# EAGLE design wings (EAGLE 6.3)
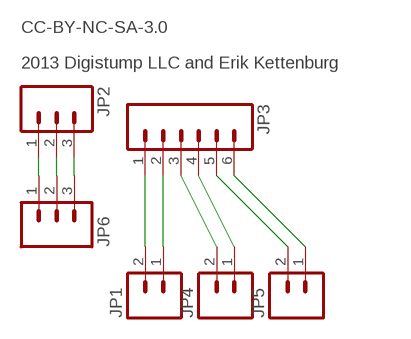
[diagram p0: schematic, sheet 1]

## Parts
JP1  M023.5MM  [SCREWTERMINAL-3.5MM-2]
JP2  M03PTH  [1X03]
JP3  M06SIP  [1X06]
JP4  M023.5MM  [SCREWTERMINAL-3.5MM-2]
JP5  M023.5MM  [SCREWTERMINAL-3.5MM-2]
JP6  M03SCREW  [SCREWTERMINAL-3.5MM-3]

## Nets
N$1: JP1.1 JP3.2
N$2: JP1.2 JP3.1
N$3: JP3.4 JP4.1
N$4: JP3.3 JP4.2
N$5: JP3.6 JP5.1
N$6: JP3.5 JP5.2
N$7: JP2.1 JP6.1
N$8: JP2.2 JP6.2
N$9: JP2.3 JP6.3

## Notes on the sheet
- CC-BY-NC-SA-3.0
- 2013 Digistump LLC and Erik Kettenburg

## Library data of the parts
JP1 JP4 JP5 = SparkFun:M02: Header 2
JP2 JP6 = SparkFun:M03: Header 3 Standard 3-pin 0.1" header. Use with straight break away headers (SKU : PRT-00116), right angle break away headers (PRT-00553), swiss pins (PRT-00743), machine pins (PRT-00117), and female headers (PRT-00115). Molex polarized connector foot print use with SKU : PRT-08232 with associated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
JP3 = SparkFun:M06: Header 6 Standard 6-pin 0.1" header. Use with straight break away headers (SKU : PRT-00116), right angle break away headers (PRT-00553), swiss pins (PRT-00743), machine pins (PRT-00117), and female headers (PRT-00115). Molex polarized connector foot print use with SKU : PRT-08094 with associated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

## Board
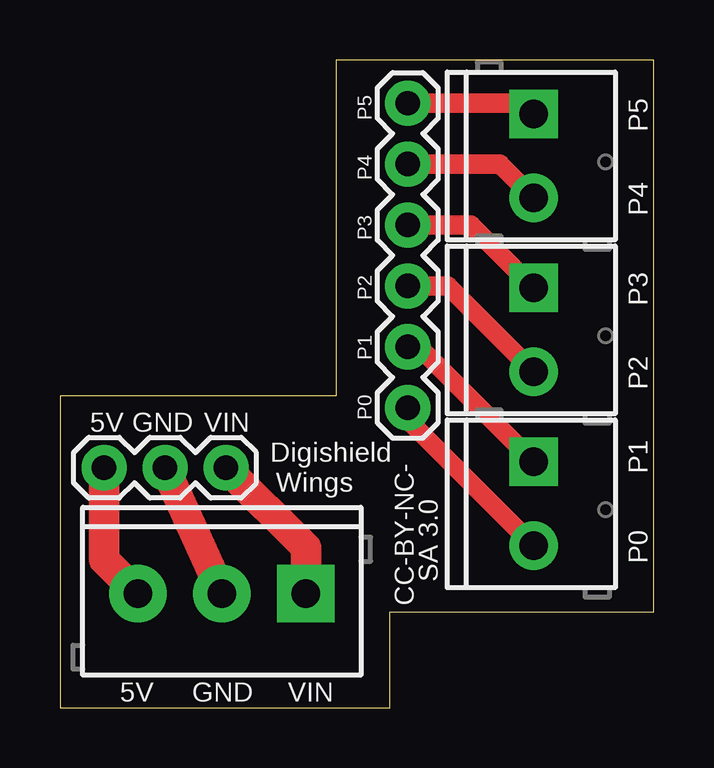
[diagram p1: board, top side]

Size 24.75 x 27 mm. Coordinates in mm from the lower left corner, seen from the top.
Outline: 11.5,27 11.5,13 0,13 0,0 13.75,0 13.75,4 24.75,4 24.75,27 11.5,27
Copper layers (1*16): Top 0.0356mm / dielectric 1.5011mm / Bottom 0.0356mm
Design rules "default": minimum track width 8mil, minimum drill 13mil, track to track 12mil, track to pad 12mil, pad to pad 12mil, via to via 12mil, smd to smd 8mil, copper to edge 15mil, drill to drill 12mil, minimum pad ring 7mil, minimum via ring 7mil, stop-mask expansion 4mil, vias tented up to drill 0mil, thermal gap 10mil

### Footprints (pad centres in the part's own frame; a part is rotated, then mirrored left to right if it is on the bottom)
SCREWTERMINAL-3.5MM-2 = drill 1.2 pad 2.032 square: 1 0,0 | drill 1.2 pad 2.032: 2 3.5,0
1X03 = drill 1.016 pad 1.88: 1 0,0; 2 2.54,0; 3 5.08,0
1X06 = drill 1.016 pad 1.88: 1 0,0; 2 2.54,0; 3 5.08,0; 4 7.62,0; 5 10.16,0; 6 12.7,0
SCREWTERMINAL-3.5MM-3 = drill 1.2 pad 2.413 square: 1 0,0 | drill 1.2 pad 2.413: 2 3.5,0; 3 7,0

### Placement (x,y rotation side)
JP1  19.75,10.25 270 top
JP2  6.92,10 180 top
JP3  14.5,12.5 90 top
JP4  19.75,17.5 270 top
JP5  19.75,24.75 270 top
JP6  10.25,4.75 180 top

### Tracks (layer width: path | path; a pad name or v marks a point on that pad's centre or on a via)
N$1
  Top 0.813: JP3.2 14.96,15.04 JP1.1
N$2
  Top 0.813: JP3.1 14.5,12 JP1.2
N$3
  Top 0.813: JP3.4 17.13,20.12 JP4.1
N$4
  Top 0.813: JP3.3 16.17,17.58 JP4.2
N$5
  Top 0.813: JP3.6 19.3,25.2 JP5.1
N$6
  Top 0.813: JP3.5 18.34,22.66 JP5.2
N$7
  Top 1.27: JP6.1 10.25,6.67 JP2.1
N$8
  Top 1.27: JP6.2 JP2.2
N$9
  Top 1.27: JP6.3 1.84,6.16 JP2.3

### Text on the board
tPlace: P5 | P4 | P3 | P2 | 5V | GND | VIN | Digishield | P1 | Wings | P0 | SA 3.0 | CC-BY-NC- | 5V | GND | VIN
tNames: P5 | P4 | P3 | P2 | P1 | P0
